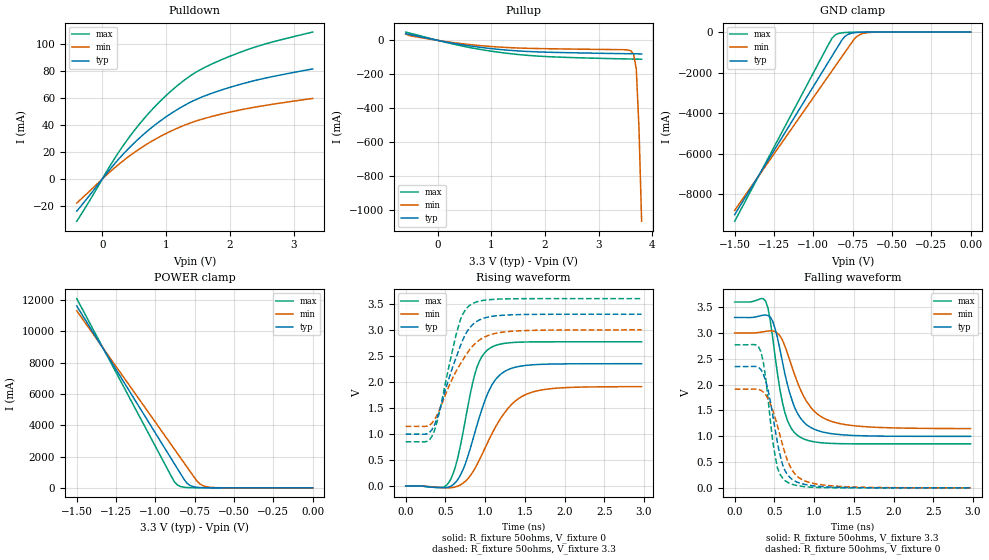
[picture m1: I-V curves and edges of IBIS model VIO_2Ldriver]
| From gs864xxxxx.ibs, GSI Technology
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|  signals   DQA1-DQA9, DQB1-DQB9, DQC1-DQC9, DQD1-DQD9
[Model]   VIO_2Ldriver
Model_type   I/O
Polarity   Non-Inverting
Vinl  =   0.8v
Vinh  =   2.0v
Vmeas =   1.5v
Cref  =   0pF
Rref  =   50
Vref  =   1.5v
|  variable   typ   min   max
C_comp   3.0pF   2.5pF   3.5pF
|  variable   typ   min   max
[Temperature Range]   50   0   100
|  variable   typ   min   max
[Voltage Range]   3.3   3.0   3.6
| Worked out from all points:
|   slope of the pulldown table from 0 to 0.495 V, typ, clamps not added: 18.7 ohm
|   slope of the pullup table from 0 to 0.495 V, typ, clamps not added: 17.8 ohm
|   GND clamp passes 1 mA (typ) near -0.58 V on its own axis
|   POWER clamp passes 1 mA (typ) near -0.61 V on its own axis
|   rising waveform, R_fixture 50ohms, V_fixture 0: 20-80 % time 304ps typ, 422ps min, 227ps max; typ from 0 V to 2.35 V
|   rising waveform, R_fixture 50ohms, V_fixture 3.3: 20-80 % time 302ps typ, 370ps min, 240ps max; typ from 0.997 V to 3.3 V
|   falling waveform, R_fixture 50ohms, V_fixture 3.3: 20-80 % time 238ps typ, 322ps min, 179ps max; typ from 3.3 V to 0.998 V
|   falling waveform, R_fixture 50ohms, V_fixture 0: 20-80 % time 176ps typ, 236ps min, 136ps max; typ from 2.35 V to 0 V
[Pulldown]
| voltage   I(typ)   I(min)   I(max)
-400mV    -23.82mA   -17.86mA   -31.34mA
-200mV    -12.17mA   -9.024mA   -16.18mA
150mV     8.912mA    6.533mA    11.97mA
450mV     24.42mA    17.92mA    32.75mA
800mV     39.14mA    28.71mA    52.49mA
1V        46.14mA    33.8mA     61.92mA
1.2V      52.23mA    38.19mA    70.16mA
1.4V      57.42mA    41.9mA     77.2mA
1.55V     60.63mA    44.22mA    81.43mA
2.05V     68.71mA    50.17mA    92.02mA
2.55V     74.83mA    54.59mA    100.2mA
3.3V      81.72mA    59.83mA    109.1mA
[Pullup]
| voltage (VDDQ-Vout)  I(typ)   I(min)   I(max)
-600mV    39.7mA     38.09mA    49.18mA
-500mV    32.74mA    26.1mA     40.9mA
250mV     -15.04mA   -11.49mA   -19.29mA
750mV     -39.34mA   -29.54mA   -51.17mA
1.3V      -57.65mA   -42.2mA    -76.49mA
2.1V      -70.15mA   -49.38mA   -96.6mA
3.45V     -78.19mA   -54.87mA   -109mA
3.6V      -78.88mA   -61.76mA   -110mA
3.65V     -79.11mA   -81.4mA    -110.3mA
3.7V      -79.35mA   -166.5mA   -110.6mA
3.75V     -79.61mA   -511.3mA   -110.9mA
3.8V      -79.96mA   -1.067A    -111.3mA
[GND Clamp]
| voltage   I(typ)   I(min)   I(max)
-1.5V     -9.007A    -8.796A    -9.334A
-900mV    -1.426A    -2.122A    -562.9mA
-880mV    -1.174A    -1.9A      -292.9mA
-860mV    -921.1mA   -1.678A    -142.5mA
-820mV    -416.2mA   -1.233A    -38.58mA
-800mV    -222mA     -1.011A    -23.51mA
-780mV    -116.3mA   -788.8mA   -16.2mA
-740mV    -33.04mA   -348.7mA   -9.876mA
-720mV    -18.57mA   -198.2mA   -8.142mA
-680mV    -6.87mA    -61.92mA   -5.539mA
-580mV    -1.002mA   -3.885mA   -1.438mA
0V        -672.8pA   -1.102nA   -625.8pA
[POWER Clamp]
| voltage (VDDQ-Vout) I(typ)   I(min)   I(max)
-1.5V     11.62A     11.31A     12.09A
-900mV    1.877A     2.768A     763.5mA
-880mV    1.553A     2.483A     398.4mA
-860mV    1.228A     2.198A     183.4mA
-840mV    903.6mA    1.913A     83.63mA
-800mV    304.2mA    1.344A     19.43mA
-780mV    154.7mA    1.059A     10.68mA
-740mV    39.51mA    489.9mA    4.639mA
-720mV    20.32mA    274.5mA    3.532mA
-680mV    5.894mA    82.85mA    2.298mA
-580mV    568.7uA    4.201mA    684.1uA
0V        1.011nA    2.697nA    667pA
[Ramp]
| voltage   typ   min   max
dV/dt_r   0.97/129p   0.8/165p   1.18/100p
dV/dt_f   0.96/128p   0.79/162p   1.17/99p
R_load  =   50ohms
[Rising Waveform]
C_fixture =   0.0pf
R_fixture =   50ohms
V_fixture =   0
| Time   V(typ)   V(min)   V(max)
0s        8.184nV    16.82nV    6.034nV
540ps     -19.75mV   -33.7mV    62.85mV
630ps     74.54mV    -14.87mV   394.5mV
720ps     308.9mV    53.95mV    1.016V
840ps     864.6mV    259.5mV    1.963V
900ps     1.184V     418.6mV    2.296V
1.08ns    1.927V     987.9mV    2.666V
1.32ns    2.255V     1.547V     2.754V
1.59ns    2.328V     1.803V     2.768V
2.97ns    2.35V      1.91V      2.771V
[Rising Waveform]
C_fixture =   0.0pf
R_fixture =   50ohms
V_fixture =   3.3
V_fixture_min =   3.0
V_fixture_max =   3.6
| Time   V(typ)   V(min)   V(max)
0s        997.4mV    1.146V     850.5mV
240ps     996.3mV    1.145V     849mV
330ps     1.082V     1.207V     953.5mV
420ps     1.424V     1.446V     1.395V
600ps     2.326V     2.103V     2.681V
690ps     2.699V     2.35V      3.204V
840ps     3.097V     2.685V     3.503V
1.02ns    3.24V      2.881V     3.575V
1.29ns    3.286V     2.968V     3.596V
2.97ns    3.3V       3V         3.6V
[Falling Waveform]
C_fixture =   0.0pf
R_fixture =   50ohms
V_fixture =   3.3
V_fixture_min =   3.0
V_fixture_max =   3.6
| Time   V(typ)   V(min)   V(max)
0s        3.3V       3V         3.6V
390ps     3.348V     3.031V     3.617V
420ps     3.339V     3.038V     3.479V
480ps     3.225V     3.038V     2.894V
570ps     2.68V      2.947V     1.9V
630ps     2.224V     2.755V     1.47V
810ps     1.393V     1.969V     995.2mV
1.02ns    1.123V     1.458V     886.4mV
1.29ns    1.037V     1.256V     857.2mV
2.97ns    997.5mV    1.148V     850.6mV
[Falling Waveform]
C_fixture =   0.0pf
R_fixture =   50ohms
V_fixture =   0
| Time   V(typ)   V(min)   V(max)
0s        2.35V      1.911V     2.771V
330ps     2.293V     1.89V      2.639V
360ps     2.209V     1.855V     2.441V
420ps     1.901V     1.728V     1.728V
480ps     1.401V     1.5V       889.1mV
540ps     855.1mV    1.192V     376.9mV
660ps     266.5mV    548.3mV    112.5mV
810ps     97.13mV    195.2mV    36.66mV
1.05ns    30.12mV    69mV       6.651mV
2.97ns    4.456uV    188.7uV    -156.3nV
